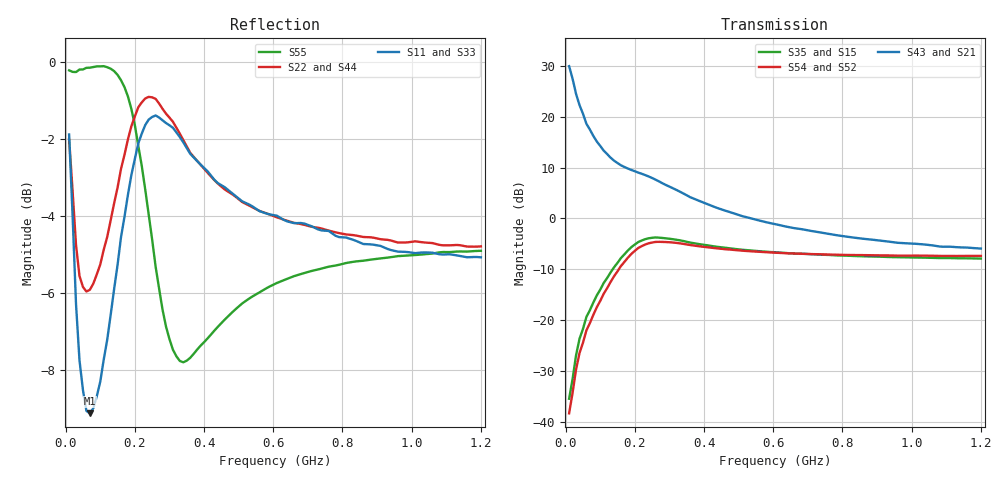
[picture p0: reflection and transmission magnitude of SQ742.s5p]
!  POLYFET RF DEVICES
!  SQ742 (EACH SIDE)
!  S PARAMETERS
!  VDS=50V, IDQ=300mA
!AWR Design Environment (2053) Wed Feb 04 15:39:43 2004
!freq-unit  param-type  data-format  keyword  impedance-ohms
# MHz  S  MA  R  50
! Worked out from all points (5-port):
!   120 points, 10 MHz to 1.2 GHz, reference 50 ohm
!   strongest paths, dB at 10 MHz, 310 MHz, 610 MHz, 910 MHz, 1.2 GHz:
!     S43: 29.9, 5.9, -1.2, -4.4, -5.9
!     S21: 29.9, 5.9, -1.2, -4.4, -5.9
!     S54: -38.2, -4.7, -6.7, -7.2, -7.3
!     S52: -38.2, -4.7, -6.7, -7.2, -7.3
!     S35: -35.4, -4.1, -6.6, -7.5, -7.9
!     S15: -35.4, -4.1, -6.6, -7.5, -7.9
!   lowest |S11| = -9.1 dB at 70 MHz (marker M1), VSWR 2.07, Z = 52.8 - j38.2 ohm
!   |S11| at or under -10 dB: nowhere
